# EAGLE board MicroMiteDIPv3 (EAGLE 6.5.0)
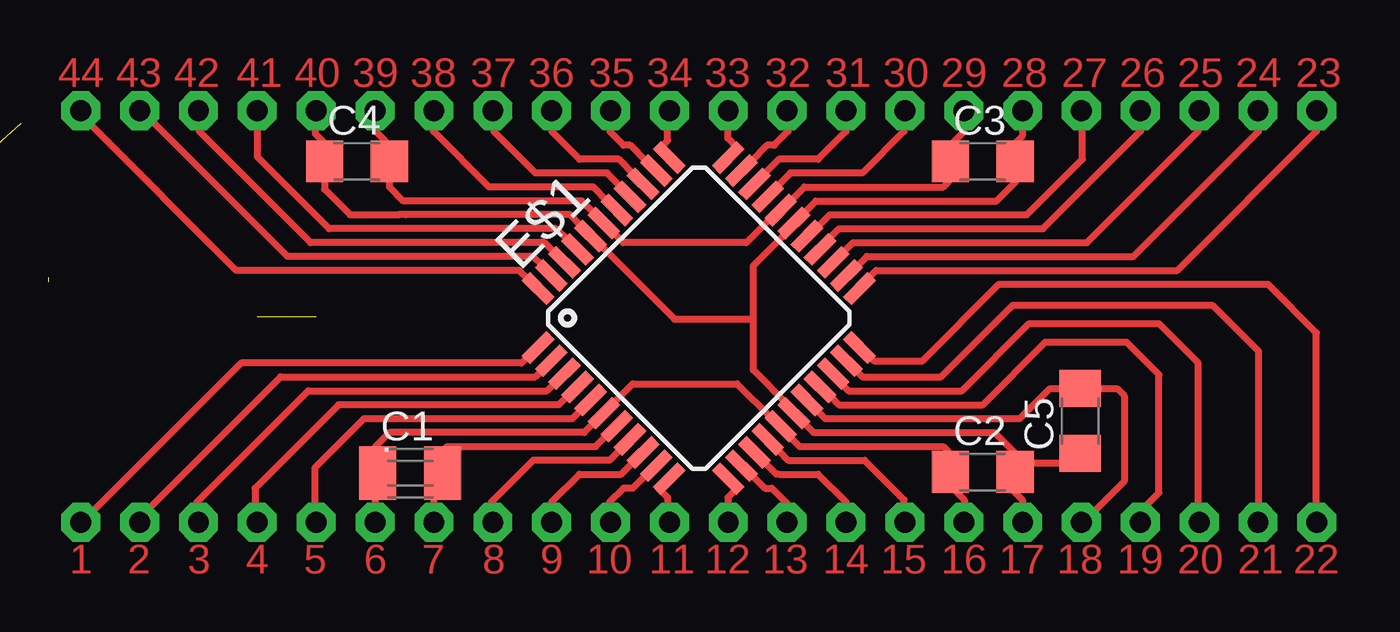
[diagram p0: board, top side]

No outline drawn. Coordinates in mm, seen from the top.
Copper layers (1*16): Top 0.035mm / dielectric 1.5mm / Bottom 0.035mm
Design rules "default": minimum track width 10mil, minimum drill 24mil, track to track 8mil, track to pad 8mil, pad to pad 8mil, via to via 8mil, smd to smd 8mil, copper to edge 40mil, drill to drill 8mil, minimum pad ring 10mil, minimum via ring 8mil, stop-mask expansion 4mil, vias tented up to drill 0mil, thermal gap 10mil

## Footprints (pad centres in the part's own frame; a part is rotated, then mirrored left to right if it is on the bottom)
C1206 = smd 1.6 x 1.8: 1 -1.4,0; 2 1.4,0
TQFP44 = smd 1.5 x 0.5: 1 -5.8,4; 2 -5.8,3.2; 3 -5.8,2.4; 4 -5.8,1.6; 5 -5.8,0.8; 6 -5.8,0; 7 -5.8,-0.8; 8 -5.8,-1.6; 9 -5.8,-2.4; 10 -5.8,-3.2; 11 -5.8,-4; 23 5.8,-4; 24 5.8,-3.2; 25 5.8,-2.4; 26 5.8,-1.6; 27 5.8,-0.8; 28 5.8,0; 29 5.8,0.8; 30 5.8,1.6; 31 5.8,2.4; 32 5.8,3.2; 33 5.8,4 | smd 0.5 x 1.5: 12 -4,-5.8; 13 -3.2,-5.8; 14 -2.4,-5.8; 15 -1.6,-5.8; 16 -0.8,-5.8; 17 0,-5.8; 18 0.8,-5.8; 19 1.6,-5.8; 20 2.4,-5.8; 21 3.2,-5.8; 22 4,-5.8; 34 4,5.8; 35 3.2,5.8; 36 2.4,5.8; 37 1.6,5.8; 38 0.8,5.8; 39 0,5.8; 40 -0.8,5.8; 41 -1.6,5.8; 42 -2.4,5.8; 43 -3.2,5.8; 44 -4,5.8

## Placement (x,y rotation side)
.  [C1206]  44.7,47.6 0 top
C1  47uF  [C1206]  44.7,48.1 0 top
C2  100nF  [C1206]  69.4,47.9 0 top
C3  100nF  [C1206]  69.4,61.3 0 top
C4  100nF  [C1206]  42.4,61.3 0 top
C5  100nF  [C1206]  73.6,50.1 90 top
E$1  [TQFP44]  57.15,54.54 45 top

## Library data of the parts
. C1-C5 = resistor
E$1 = microchip

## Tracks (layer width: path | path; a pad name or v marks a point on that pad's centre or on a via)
S$1
  Top 0.305: 83.8,62.9 83.8,62.6 77.8,56.6 64.8,56.6 63.8,55.6
S$2
  Top 0.305: 76.2,62.9 76.2,62.6 72,58.4 63.2,58.4 62.2,57.4
S$3
  Top 0.305: 64.4,53 64.7,52.7 66.8,52.7 70.1,56 81.7,56 83.8,53.9 83.8,46.4
S$4
  Top 0.305: 63.4,56.2 64.4,57.2 75.9,57.2 81.3,62.6 81.3,62.8
S$5
  Top 0.305: 63.5,62.8 63.5,62.6 62.3,61.4 60.6,61.4 59.4,60.2
S$6
  Top 0.305: 61.1,49.4 61.5,49 67.7,49 68.1,48.6
S$7  (via drill 0.9 pad 1.68)
  other vias: 58.42,45.72
S$8
  Top 0.305: 63.8,52.4 64.2,52 67.6,52 67.7,52.1 67.8,52.2 70.7,55.1 79.3,55.1 81.3,53.1 81.3,46.4
S$10
  Top 0.305: 62.8,51.2 63.2,50.8 69.4,50.8 72.1,53.5 75.6,53.5 77,52.1 77,47 76.4,46.4
S$11
  Top 0.305: 62.2,50.6 62.6,50.2 71,50.2 72.3,51.5 75.2,51.5 75.5,51.2 75.5,47.5 74.1,46.1
S$12
  Top 0.305: 60.6,48.8 61,48.4 64.3,48.4 66,46.7 66,46.4
S$13
  Top 0.305: 60.6,47.8 62.3,47.8 63.5,46.6 63.5,46.5
S$14
  Top 0.305: 61,46.4 61,46.5 60.3,47.2 60,47.2 59.4,47.8
S$15  (via drill 0.9 pad 1.68)
  other vias: 66.04,45.72
S$16
  Top 0.305: 61.1,59.6 61.7,60.2 67.7,60.2 68.1,60.6
S$17
  Top 0.305: 61.6,57.8 62.8,59 71.3,59 73.7,61.4 73.7,62.9
S$18
  Top 0.305: 61,58.4 62.2,59.6 70,59.6 70.8,60.4 70.8,60.6 70.7,60.7
S$19
  Top 0.305: 59.4,61.3 60.1,62 60.4,62 61,62.6 61,62.8
S$20
  Top 0.305: 78.7,46.4 78.7,52.6 77,54.3 71.4,54.3 68.5,51.4 63.6,51.4 63.2,51.8
S$21
  Top 0.305: 60.5,60.2 61.1,60.8 64.2,60.8 66,62.6 66,62.8
S$22
  Top 0.305: 78.7,62.8 78.7,62.6 73.9,57.8 63.8,57.8 62.8,56.8
S$23
  Top 0.305: 58.8,61.9 58.4,62.3 58.4,62.9
S$24
  Top 0.305: 55.5,61.9 55.8,62.2 55.8,62.8
S$25
  Top 0.305: 53.3,62.7 53.3,62.6 53.9,62 54.2,62 54.9,61.3
S$26
  Top 0.305: 50.8,62.7 50.8,62.6 52,61.4 53.7,61.4 54.4,60.7
S$27
  Top 0.305: 48.3,62.7 48.3,62.6 50.1,60.8 53.2,60.8 53.8,60.2
S$28  (via drill 0.9 pad 1.68)
  other vias: 60.96,63.5
S$29
  Top 0.305: 45.7,62.8 45.7,62.6 48.1,60.2 52.6,60.2 53.2,59.6
S$30
  Top 0.305: 52.6,59.1 52.1,59.6 44.4,59.6 43.8,60.2 43.8,60.7
S$31
  Top 0.305: 43.2,62.8 43.2,62.6 44,61.8
S$32
  Top 0.305: 51.5,57.9 51,58.4 41.2,58.4 38.1,61.5 38.1,62.8
S$33
  Top 0.305: 35.6,62.7 35.6,62.6 40.4,57.8 50.5,57.8 50.9,57.4
S$34
  Top 0.305: 50.4,56.8 50,57.2 39.4,57.2 33.6,63
S$35
  Top 0.305: 71.4,48.3 73.3,48.3
S$36
  Top 0.305: 52.1,50.6 51.7,50.2 42.7,50.2 40.6,48.1 40.6,46.4
S$37
  Top 0.305: 52.7,50.1 52.2,49.6 43.8,49.6 43.2,49 43.2,46.4
S$38  (via drill 0.9 pad 1.68)
  other vias: 63.5,63.5
S$39  (via drill 0.9 pad 1.68)
  other vias: 66.04,63.5
S$40  (via drill 0.9 pad 1.68)
  other vias: 68.58,63.5
S$41  (via drill 0.9 pad 1.68)
  other vias: 71.12,63.5
S$42  (via drill 0.9 pad 1.68)
  other vias: 73.66,63.5
S$43  (via drill 0.9 pad 1.68)
  other vias: 76.2,63.5
S$44  (via drill 0.9 pad 1.68)
  other vias: 78.74,63.5
S$45  (via drill 0.9 pad 1.68)
  other vias: 81.28,63.5
S$46  (via drill 0.9 pad 1.68)
  other vias: 83.82,63.5
S$47  (via drill 0.9 pad 1.68)
  other vias: 58.42,63.5
S$48  (via drill 0.9 pad 1.68)
  other vias: 55.88,63.5
S$49  (via drill 0.9 pad 1.68)
  other vias: 53.34,63.5
S$50  (via drill 0.9 pad 1.68)
  other vias: 50.8,63.5
S$51  (via drill 0.9 pad 1.68)
  other vias: 48.26,63.5
S$52  (via drill 0.9 pad 1.68)
  other vias: 45.72,63.5
S$53  (via drill 0.9 pad 1.68)
  other vias: 43.18,63.5
S$54  (via drill 0.9 pad 1.68)
  other vias: 40.64,63.5
S$55  (via drill 0.9 pad 1.68)
  other vias: 38.1,63.5
S$56  (via drill 0.9 pad 1.68)
  other vias: 35.56,63.5
S$57  (via drill 0.9 pad 1.68)
  other vias: 33.02,63.5
S$58  (via drill 0.9 pad 1.68)
  other vias: 30.48,63.5
S$59  (via drill 0.9 pad 1.68)
  other vias: 55.88,45.72
S$60  (via drill 0.9 pad 1.68)
  other vias: 53.34,45.72
S$61  (via drill 0.9 pad 1.68)
  other vias: 50.8,45.72
S$62  (via drill 0.9 pad 1.68)
  other vias: 48.26,45.72
S$63  (via drill 0.9 pad 1.68)
  other vias: 45.72,45.72
S$64  (via drill 0.9 pad 1.68)
  other vias: 43.18,45.72
S$65  (via drill 0.9 pad 1.68)
  other vias: 40.64,45.72
S$66  (via drill 0.9 pad 1.68)
  other vias: 38.1,45.72
S$67  (via drill 0.9 pad 1.68)
  other vias: 35.56,45.72
S$68  (via drill 0.9 pad 1.68)
  other vias: 33.02,45.72
S$69  (via drill 0.9 pad 1.68)
  other vias: 30.48,45.72
S$70  (via drill 0.9 pad 1.68)
  other vias: 60.96,45.72
S$71  (via drill 0.9 pad 1.68)
  other vias: 63.5,45.72
S$72  (via drill 0.9 pad 1.68)
  other vias: 68.58,45.72
S$73  (via drill 0.9 pad 1.68)
  other vias: 71.12,45.72
S$74  (via drill 0.9 pad 1.68)
  other vias: 73.66,45.72
S$75  (via drill 0.9 pad 1.68)
  other vias: 76.2,45.72
S$76  (via drill 0.9 pad 1.68)
  other vias: 78.74,45.72
S$77  (via drill 0.9 pad 1.68)
  other vias: 81.28,45.72
S$78  (via drill 0.9 pad 1.68)
  other vias: 83.82,45.72
S$79
  Top 0.305: 60.5,47.8 59.9,48.4
S$87
  Top 0.305: 68.6,62.8 68.6,62.6 67.9,61.9
S$88
  Top 0.305: 58.8,47.2 58.4,46.8 58.4,46.4
S$89
  Top 0.305: 55.4,47.2 55.8,46.8 55.8,46.4
S$90
  Top 0.305: 53.2,49.5 52.7,49 46.3,49 45.7,48.4 45.7,46.5
S$91
  Top 0.305: 50.8,46.3 50.8,46.6 52,47.8 53.8,47.8 54.4,48.4
S$92
  Top 0.305: 48.2,46.4 48.2,46.6 50,48.4 53.3,48.4 53.8,48.9
S$94
  Top 0.305: 50.4,52.3 50.1,52 39.1,52 33.5,46.4
S$95
  Top 0.305: 68.6,46.4 68.6,46.7 67.8,47.5
S$96
  Top 0.305: 70.8,48.7 69.9,49.6 62.1,49.6 61.7,50
S$97
  Top 0.305: 71.1,46.5 71.1,46.7 70.7,47.1
S$98
  Top 0.305: 71.1,62.8 71.1,62.4 70.8,62.1
S$99
  Top 0.305: 35.5,46.5 35.5,46.6 40.3,51.4 50.6,51.4 51,51.8
S$100
  Top 0.305: 53.3,46.4 53.3,46.6 53.9,47.2 54.3,47.2 54.9,47.8
S$107
  Top 0.305: 60.2,58.8 59.2,57.8 53.9,57.8 53.4,58.3
S$108
  Top 0.305: 40.6,62.8 40.6,62.5 41,62.1
S$109
  Top 0.305: 60.3,50.2 58.8,51.7 54.3,51.7 53.5,50.9
S$110
  Top 0.305: 41,60.5 41,60.1 42.1,59 44.2,59 44.5,59 51.6,59 52.1,58.5
S$113  (1 unrouted)
S$121  (1 unrouted)
S$122  (2 unrouted)
S$125
  Top 0.305: 49.8,56.2 49.4,56.6 37.2,56.6 30.8,63
S$135  (1 unrouted)
S$136
  Top 0.305: 52.9,57.7 56.1,54.5 59.5,54.5 | 60.9,58.2 59.5,56.8 59.5,54.5 | 61,50.8 59.5,52.3 59.5,54.5
S$137
  Top 0.305: 49.8,52.9 49.5,52.6 37.4,52.6 31,46.2
S$147
  Top 0.305: 38,46.4 38,47.2 41.6,50.8 51.1,50.8 51.5,51.2

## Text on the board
Top: 44 | 43 | 42 | 41 | 40 | 39 | 38 | 37 | 36 | 35 | 34 | 33 | 32 | 31 | 30 | 29 | 28 | 27 | 26 | 25 | 24 | 23 | 1 | 2 | 3 | 4 | 5 | 6 | 7 | 8 | 9 | 10 | 11 | 12 | 13 | 14 | 15 | 16 | 17 | 18 | 19 | 20 | 21 | 22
